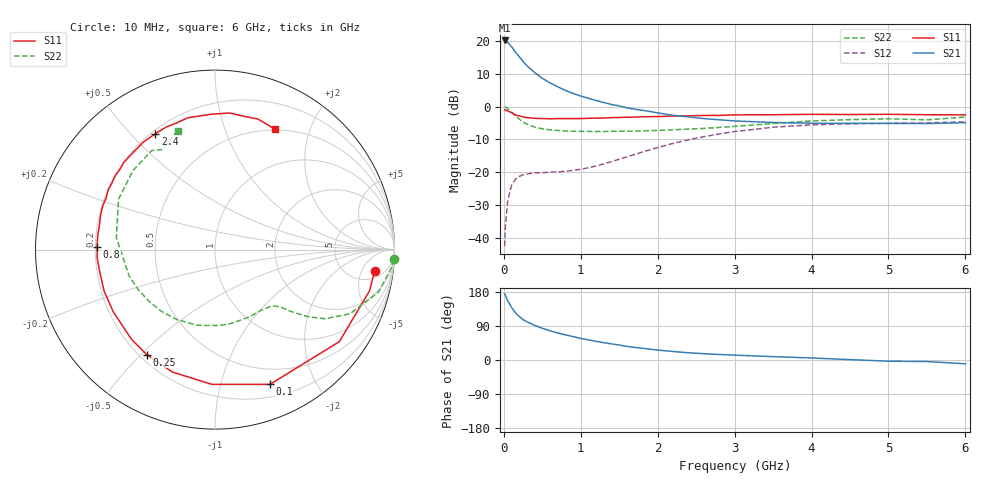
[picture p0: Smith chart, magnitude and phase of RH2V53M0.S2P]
! SIEMENS Small Signal Semiconductors
! BFR106
! Si NPN RF Bipolar Junction Transistor in SOT23
! VCE = 2.5 V  IC = 3 mA
! Common Emitter S-Parameters:  August  1996
# GHz  S  MA  R  50
!  f  S11  S21  S12  S22
! GHz  MAG  ANG  MAG  ANG  MAG  ANG  MAG  ANG
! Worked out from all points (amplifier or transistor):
!   36 points, 10 MHz to 6 GHz, reference 50 ohm
!   highest |S21| = 20.2 dB at 10 MHz (marker M1)
!   |S21| within 3 dB of that: start of sweep to 134 MHz
!   unconditionally stable (mu >= 1): 708.4 MHz to 2.105 GHz; 3.97 GHz to end of sweep
!   at 250 MHz: K = 0.39, MSG = 17.3 dB, |S12| = -20.8 dB
!   at 1.4 GHz: K = 1.23, MAG = 5.9 dB, |S12| = -16.8 dB
!   at 6 GHz: K = 1.02, MAG = -1.1 dB, |S12| = -4.6 dB
!   S11 on the Smith chart (normalised r, x): 10 MHz: 7, -9; 100 MHz: 0.33, -1.44; 250 MHz: 0.23, -0.52; 800 MHz: 0.21, +0.01; 2.4 GHz: 0.22, +0.59; 6 GHz: 0.49, +1.50
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0.01  0.8967 -7.6  10.29 174.6  0.0074 85.8  0.9962 -3.1
0.02  0.8913 -14.9  10.19 170.6  0.0149 82.1  0.9864 -6.2
0.05  0.862 -36.5  9.546 156.7  0.0362 71.1  0.9411 -14.6
0.1  0.8108 -67.8  8.289 139.0  0.0624 56.2  0.8335 -25.4
0.15  0.751 -91.3  6.854 124.5  0.0776 45.1  0.7256 -32.1
0.2  0.7224 -109.2  5.804 114.8  0.0862 39.0  0.646 -35.5
0.25  0.6977 -123.1  4.927 106.5  0.0911 34.5  0.5815 -37.8
0.3  0.6824 -133.1  4.238 100.8  0.094 32.3  0.5421 -39.3
0.4  0.6643 -148.7  3.328 91.5  0.0975 29.6  0.489 -41.1
0.5  0.6595 -159.6  2.719 83.7  0.0983 29.4  0.4591 -43.1
0.6  0.654 -168.4  2.315 77.1  0.0999 31.0  0.443 -45.8
0.8  0.6575 178.7  1.777 66.4  0.1037 36.5  0.4253 -52.3
1.1  0.6662 163.0  1.344 53.0  0.1168 47.6  0.4196 -64.2
1.6  0.6917 143.5  0.963 36.0  0.1714 60.1  0.4232 -87.5
2.2  0.7197 123.6  0.739 22.4  0.2751 58.8  0.4443 -119.0
2.4  0.7261 117.3  0.699 19.1  0.3129 56.0  0.4554 -130.8
3  0.7499 101.7  0.606 12.8  0.4175 44.4  0.5004 -162.8
3.5  0.7545 91.8  0.574 8.9  0.4859 33.6  0.5536 173.2
4.5  0.7599 77.5  0.557 1.0  0.5484 13.7  0.6351 135.9
5  0.7656 71.9  0.556 -3.2  0.5594 6.1  0.6548 122.5
5.5  0.7547 67.0  0.553 -4.1  0.5662 2.5  0.6303 117.9
6  0.7496 63.5  0.57 -9.9  0.589 -5.2  0.6949 107.3
